| Texas Instruments Incorporated
| Four-Port USB 3.1 Hub
| Marketing part#   Voltage Range   Package-type   Temperature
| TUSB8043RGC   2.97V - 3.465V   64-Pin RGC   0 to 70 C
[IBIS Ver]   4.1
[File name]   tusb8043rgc.ibs
[File Rev]   1.0
[Date]   05/31/2017
[Source]   Model built from TISPICE simulations at:
   Texas Instruments Incorporated.
   Analog-eLab, HPA
   12500 TI Blvd
   Dallas, TX -75243
[Notes]   Rev 1.0: 05/31/2017
   - Model based on v1.0 IBIS model for TUSB8041q1 dated 02/28/2014
[Disclaimer] This product is designed as an aid for customers of Texas Instruments.
   No warranties, either expressed or implied, with respect to this third
   party software (if any) or with respect to its fitness for any
   particular purpose is claimed by Texas Instruments or the author. The
   software (if any) is provided solely on an "as is" basis. The entire
   risk as to its quality and performance is with the customer
[Copyright]   (C)Copyright 2017 Texas Instruments Incorporated.
   All rights reserved.
|   TUSB8043
[Component]   TUSB8043
[Manufacturer]  Texas Instruments Incorporated
[Package]   |64-pin RGC
|   typ   min   max
R_pkg   0.2389   0.0142   0.3346
L_pkg   2.3741nH   1.4298nH   2.8522nH
C_pkg   0.8499pF   0.7143pF   1.0609pF
[PIN]   signal_name   model_name   R_pin   L_pin   C_pin
1   USB_DP_DN1   usb2   NA   NA   NA
2   USB_DM_DN1   usb2   NA   NA   NA
3   USB_SSTXP_DN1   usb3   NA   NA   NA
4   USB_SSTXM_DN1   usb3   NA   NA   NA
5   VDD   POWER   NA   NA   NA
6   USB_SSRXP_DN1   RXP_N   NA   NA   NA
7   USB_SSRXM_DN1   RXP_N   NA   NA   NA
8   VDD   POWER   NA   NA   NA
9   USB_DP_DN2   usb2   NA   NA   NA
10   USB_DM_DN2   usb2   NA   NA   NA
11   USB_SSTXP_DN2   usb3   NA   NA   NA
12   USB_SSTXM_DN2   usb3   NA   NA   NA
13   VDD   POWER   NA   NA   NA
14   USB_SSRXP_DN2   RXP_N   NA   NA   NA
15   USB_SSRXM_DN2   RXP_N   NA   NA   NA
16   VDD33   POWER   NA   NA   NA
17   USB_DP_DN3   usb2   NA   NA   NA
18   USB_DM_DN3   usb2   NA   NA   NA
19   USB_SSTXP_DN3   usb3   NA   NA   NA
20   USB_SSTXM_DN3   usb3   NA   NA   NA
21   VDD   POWER   NA   NA   NA
22   USB_SSRXP_DN3   RXP_N   NA   NA   NA
23   USB_SSRXM_DN3   RXP_N   NA   NA   NA
24   USB_DP_DN4   usb2   NA   NA   NA
25   USB_DM_DN4   usb2   NA   NA   NA
26   USB_SSTXP_DN4   usb3   NA   NA   NA
27   USB_SSTXM_DN4   usb3   NA   NA   NA
28   VDD   POWER   NA   NA   NA
29   USB_SSRXP_DN4   RXP_N   NA   NA   NA
30   USB_SSRXM_DN4   RXP_N   NA   NA   NA
31   VDD   POWER   NA   NA   NA
32   PWRCTL4/BATEN4   BC3340DSHYPBFZP18PD   NA   NA   NA
33   PWRCTL3/BATEN3   BC3340DSHYPBFZP18PD   NA   NA   NA
34   VDD33   POWER   NA   NA   NA
35   PWRCTL2/BATEN2   BC3340DSHYPBFZP18PD   NA   NA   NA
36   PWRCTL1/BATEN1   BC3340DSHYPBFZP18PD   NA   NA   NA
37   SDA/SMBDAT   BC3340DSHYPBFZP18PD   NA   NA   NA
38   SCL/SMBCLK   BC3340DSHYPBFZP18PD   NA   NA   NA
39   SMBUSZ/SS_SUSPEND   BC3340DSHYPBFZP18PU   NA   NA   NA
40   FULLPWRMGMT   BC3340DSHYPBFZP18PD   NA   NA   NA
41   POWCTL_POL   BC3340DSHYPBFZP18PU   NA   NA   NA
42   GANGED/SMBAS2   BC3340DSHYPBFZP18PD   NA   NA   NA
43   OVERCUR4Z   IC33SHYPBFZP18PU   NA   NA   NA
44   OVERCUR3Z   IC33SHYPBFZP18PU   NA   NA   NA
45   AUTOENZ/HS_SUSPEND   BC3340DSHYPBFZP18PU   NA   NA   NA
46   OVERCUR1Z   IC33SHYPBFZP18PU   NA   NA   NA
47   OVERCUR2Z   IC33SHYPBFZP18PU   NA   NA   NA
48   USB_VBUS   IC33SHYPBFZP18   NA   NA   NA
49   TEST   IC33SHYPBFZP18PD   NA   NA   NA
50   GRSTZ   IC33SHYPBFZP18PU   NA   NA   NA
51   VDD   POWER   NA   NA   NA
52   VDD33   POWER   NA   NA   NA
53   USB_DP_UP   usb2   NA   NA   NA
54   USB_DM_UP   usb2   NA   NA   NA
55   USB_SSTXP_UP   usb3   NA   NA   NA
56   USB_SSTXM_UP   usb3   NA   NA   NA
57   VDD   POWER   NA   NA   NA
58   USB_SSRXP_UP   RXP_N   NA   NA   NA
59   USB_SSRXM_UP   RXP_N   NA   NA   NA
60   NC   NC   NA   NA   NA
61   XO   NC   NA   NA   NA
62   XI   NC   NA   NA   NA
63   VDD33   POWER   NA   NA   NA
64   USB_R1   NC   NA   NA   NA
[Diff_pin]   inv_pin   vdiff   tdelay_typ   tdelay_min   tdelay_max
1   2   NA   NA   NA   NA
3   4   NA   NA   NA   NA
6   7   200mV   NA   NA   NA
9   10   NA   NA   NA   NA
11   12   NA   NA   NA   NA
14   15   200mV   NA   NA   NA
17   18   NA   NA   NA   NA
19   20   NA   NA   NA   NA
22   23   200mV   NA   NA   NA
24   25   NA   NA   NA   NA
26   27   NA   NA   NA   NA
29   30   200mV   NA   NA   NA
53   54   NA   NA   NA   NA
55   56   NA   NA   NA   NA
58   59   200mV   NA   NA   NA
[Model Selector] usb2
usb2_HS_R   USB 2.0 High Speed mode, for DP/DM pin 240MHz
usb2_HS_RC   USB 2.0 High Speed mode, for DP/DM pin 240MHz, with Cfixture
usb2_FS_R   USB 2.0 Fast Speed mode, for DP/DM pin 6MHz
usb2_FS_RC   USB 2.0 Fast Speed mode, for DP/DM pin 6MHz, with Cfixture
usb2_LS_RC   USB 2.0 Low  Speed mode, for DP/DM pin 750kHz, with Cfixture
usb2_LS_R   USB 2.0 Low  Speed mode, for DP/DM pin 750kHz
[Model Selector] usb3
usb3_DE   USB 3.0 De-Emphasis mode, best at 1.25GHz
usb3_WODE   USB 3.0 No De-Emphasis mode, for SSTXP/N 2.5GHz
usb3_SATA1   USB 3.0 SATA1 mode, for SSTXP/N 750MHz
usb3_SATA2   USB 3.0 SATA2 mode, for SSTXP/N 1.5GHz
pcie_GEN2   PCI-E 2.5GHz  GEN2 model
pcie_GEN1   PCI-E 1.25GHz GEN1 model
[Model Selector] BC3340DSHYPBFZP18
HYPBFZP18_PI_5P_3P3 BUFFER WITHOUT PULLUP/PULLDOWN & 5% VDDS TOLERANCE
HYPBFZP18_PI_10P_3P3 BUFFER WITHOUT PULLUP/PULLDOWN & 10% VDDS TOLERANCE
[Model Selector] BC3340DSHYPBFZP18PU
FZP18_PU_PI_5P_3P3 BUFFER WITH WEAK PULLUP & 5% VDDS TOLERANCE
FZP18_PU_PI_10P_3P3 BUFFER WITH WEAK PULLUP & 10% VDDS TOLERANCE
[Model Selector] BC3340DSHYPBFZP18PD
FZP18_PD_PI_5P_3P3 BUFFER WITH WEAK PULLDOWN & 5% VDDS TOLERANCE
FZP18_PD_PI_10P_3P3 BUFFER WITH WEAK PULLDOWN & 10% VDDS TOLERANCE
[Model Selector] IC33SHYPBFZP18
C33SHYPBFZP18_10P BUFFER WITHOUT PULLUP/PULLDOWN & 10% VDDS TOLERANCE
C33SHYPBFZP18_5P  BUFFER WITHOUT PULLUP/PULLDOWN & 5% VDDS TOLERANCE
[Model Selector] IC33SHYPBFZP18PD
YPBFZP18_PD_5P BUFFER with WEAK PULLDOWN & 5% VDDS TOLERANCE
YPBFZP18_PD_10P BUFFER with WEAK PULLDOWN & 5% VDDS TOLERANCE
[Model Selector] IC33SHYPBFZP18PU
PBFZP18_PU_5P BUFFER with WEAK PULLUP & 5% VDDS TOLERANCE
PBFZP18_PU_10P BUFFER with WEAK PULLUP & 10% VDDS TOLERANCE
|USB 3.0 De-Emphasis mode, for SSTXP/SSTXN pins 2.5Gbps(1.25GHz to De-Emphasis)
[Model]   usb3_DE
Model_type   Output
Vmeas = 1.1
Vref = 1.1
Rref = 50
|   typ   min   max
|   (TYP PVT)   (Fast PVT) (Slow PVT)
C_comp   0pF   0pF   0pF
[Driver Schedule]
| Model_name   Rise_on_dly Rise_off_dly Fall_on_dly Fall_off_dly
usb3_de_MAIN   0.0nS   NA   0   NA
usb3_de_BOOST   NA   0.2nS   NA   0.2nS
[Voltage Range]   1.1   0.99   1.155
[Temperature Range]   27   105   -40
[Pullup Reference]   1.1   0.99   1.155
[Pulldown Reference]   0   0   0
[Power Clamp Reference]   1.1   0.99   1.155
[GND Clamp Reference]   0   0   0
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[Ramp]
R_load = 50
|   typ   min   max
dV/dt_r   0.972315/1.549e-011   0.988218/1.8606e-011   0.957162/1.40763e-011
dV/dt_f   0.972312/7.7916e-012   0.988183/1.21282e-011  0.957081/6.00194e-012
|PCIE GEN2 De-Emphasis mode, for SSTXP/SSTXN pins 5Gbps(2.5GHz to De-Emphasis)
[Model]   pcie_GEN2
Model_type   Output
Vmeas = 1.1
Vref = 1.1
Rref = 50
|   typ   min   max
|   (TYP PVT)   (Fast PVT) (Slow PVT)
C_comp   0pF   0pF   0pF
[Driver Schedule]
| Model_name   Rise_on_dly Rise_off_dly Fall_on_dly Fall_off_dly
usb3_de_MAIN   0.0nS   NA   0   NA
usb3_de_BOOST   NA   0.2nS   NA   0.2nS
[Voltage Range]   1.1   0.99   1.155
[Temperature Range]   27   105   -40
[Pullup Reference]   1.1   0.99   1.155
[Pulldown Reference]   0   0   0
[Power Clamp Reference]   1.1   0.99   1.155
[GND Clamp Reference]   0   0   0
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[Ramp]
R_load = 50
|   typ   min   max
dV/dt_r   0.972315/1.549e-011   0.988218/1.8606e-011   0.957162/1.40763e-011
dV/dt_f   0.972312/7.7916e-012   0.988183/1.21282e-011  0.957081/6.00194e-012
|PCIE GEN1 De-Emphasis mode, for SSTXP/SSTXN pins 2.5Gbps(1.25GHz to De-Emphasis)
[Model]   pcie_GEN1
Model_type   Output
Vmeas = 1.1
Vref = 1.1
Rref = 50
|   typ   min   max
|   (TYP PVT)   (Fast PVT) (Slow PVT)
C_comp   0pF   0pF   0pF
[Driver Schedule]
| Model_name   Rise_on_dly Rise_off_dly Fall_on_dly Fall_off_dly
usb3_de_MAIN   0.0nS   NA   0   NA
usb3_de_BOOST   NA   0.4nS   NA   0.4nS
[Voltage Range]   1.1   0.99   1.155
[Temperature Range]   27   105   -40
[Pullup Reference]   1.1   0.99   1.155
[Pulldown Reference]   0   0   0
[Power Clamp Reference]   1.1   0.99   1.155
[GND Clamp Reference]   0   0   0
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[Ramp]
R_load = 50
|   typ   min   max
dV/dt_r   0.972315/1.549e-011   0.988218/1.8606e-011   0.957162/1.40763e-011
dV/dt_f   0.972312/7.7916e-012   0.988183/1.21282e-011  0.957081/6.00194e-012
| Models and submodels in the file (27): RXP_N (Input), usb2_FS_R (I/O), usb2_FS_RC (I/O), usb2_HS_R (I/O), usb2_HS_RC (I/O), usb2_LS_R (I/O), usb2_LS_RC (I/O), usb3_WODE (Output), usb3_SATA1 (Output), usb3_SATA2 (Output), usb3_DE (Output), usb3_de_MAIN (Output), usb3_de_BOOST (Open_drain), pcie_GEN2 (Output), pcie_GEN1 (Output), HYPBFZP18_PI_5P_3P3 (I/O), HYPBFZP18_PI_10P_3P3 (I/O), FZP18_PU_PI_5P_3P3 (I/O), FZP18_PU_PI_10P_3P3 (I/O), FZP18_PD_PI_5P_3P3 (I/O), FZP18_PD_PI_10P_3P3 (I/O), YPBFZP18_PD_10P (Input), PBFZP18_PU_10P (Input), C33SHYPBFZP18_10P (Input), YPBFZP18_PD_5P (Input), PBFZP18_PU_5P (Input), C33SHYPBFZP18_5P (Input)
